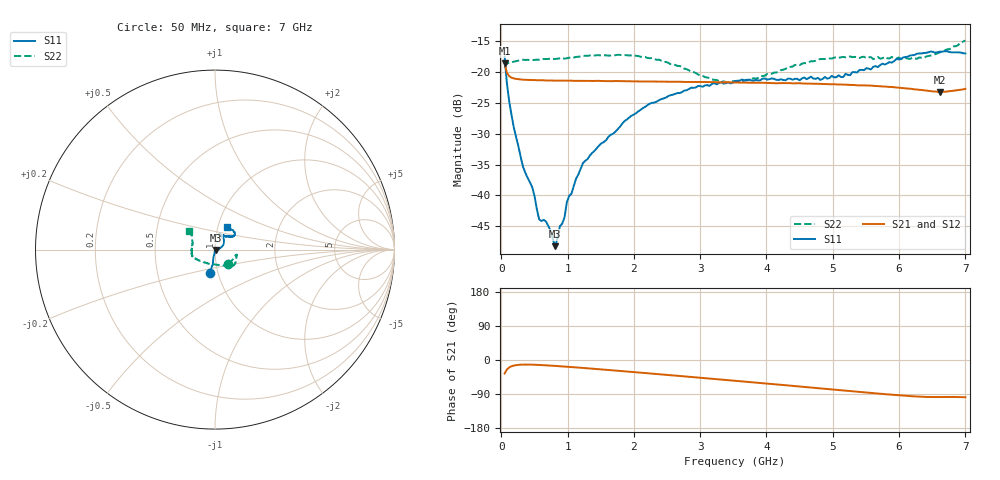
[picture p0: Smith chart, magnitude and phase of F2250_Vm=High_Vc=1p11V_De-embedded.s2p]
! Integrated Device Technology
! Corporate Headquarters
! 6024 Silver Creek Valley Road
! San Jose, CA 95138  USA
! Phone:  1-408-284-8200
! Toll Free:  1-800-223-1366
! Webpage:  http://www.idt.com/
! Timing and RF Division
! 515 Groton Road, Suite 102
! Westford, MA 01886-6024
! Device:  F2250
! Description: Voltage Variable RF Attenuator
! Frequency:  50.0 -  6000.00 MHz
! Package:  3x3 mm Thin QFN Plastic Package: 16 pin
! Ports:  2 RF, 3 DC
!  Pin  1  = GND
!  Pin  2  = NC
!  Pin  3  = RF1  = Port 1
!  Pin  4  = NC
!  Pin  5  = GND
!  Pin  6  = GND
!  Pin  7  = GND
!  Pin  8  = GND
!  Pin  9  = NC
!  Pin 10  = RF2  = Port 2
!  Pin 11  = NC
!  Pin 12  = GND
!  Pin 13  = GND
!  Pin 14  = VCNTRL
!  Pin 15  = VDD
!  Pin 16  = VMODE
! Vcntrl:  1.110 Volts
! Vmode:  +3.300 Volts
! Vdd:  +3.30  Volts
! Current:  1.329 mA
! Data:  The device was measured on a the F2250 evaluation board which has
!  individual transmission lines to the RF pins.  Data was collected
!  using a calibrated network analyzer.  The evaluation board was
!  de-embedded using a TRL calibration technique.
!  The reference plane is the edge of the package pin.
! Misc:  SN 10
!  Action Tracker AT0258
! Date Measured:  2014-11-26
! Date:  2015-10-15  MJV
! Note:
!  Integrated Device Technology supplies this data as a sample of measured
!  data at the package pin for this product.  Your particular data for this
!  product may vary.
!  Data was taken at 25 degrees C.
!  Integrated Device Technology reserves the right to change this data at anytime.
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# GHz S dB R 50
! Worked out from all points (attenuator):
!   201 points, 50 MHz to 7 GHz, reference 50 ohm
!   highest |S21| = -18.58 dB at 50 MHz (marker M1); lowest = -23.2 dB at 6.618 GHz (marker M2)
!   lowest |S11| = -48.2 dB at 814.5 MHz (marker M3), VSWR 1.01, Z = 50.3 - j0.188 ohm
!   |S11| at or under -10 dB: start of sweep to end of sweep
!   |S22| runs from -21.7 to -14.9 dB; largest |S21 - S12| = 0.00041
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0.05  -17.50 -102.6  -18.58 -35.6  -18.58 -35.6  -19.33 -47.2
0.08475  -21.87 -98.4  -20.15 -25.1  -20.14 -25.1  -18.64 -24.3
0.15425  -27.00 -101.4  -20.94 -16.6  -20.93 -16.5  -18.48 -14.7
0.328  -35.36 -98.5  -21.27 -12.1  -21.26 -12.1  -18.03 -13.0
0.467  -38.69 -98.4  -21.32 -12.3  -21.30 -12.3  -18.09 -14.8
0.57125  -43.88 -81.5  -21.35 -13.0  -21.35 -13.1  -18.03 -17.3
0.6755  -44.24 -71.6  -21.39 -14.0  -21.37 -14.0  -17.92 -19.2
0.8145  -48.21 -28.7  -21.42 -15.6  -21.40 -15.6  -17.90 -22.8
0.884  -44.97 -20.2  -21.41 -16.4  -21.41 -16.4  -17.82 -25.0
0.9535  -43.55 -28.2  -21.42 -17.3  -21.42 -17.3  -17.85 -26.1
0.98825  -41.12 -21.4  -21.42 -17.7  -21.43 -17.7  -17.80 -26.8
1.2315  -34.78 2.6  -21.45 -20.9  -21.45 -20.9  -17.40 -31.4
1.857  -27.98 22.0  -21.50 -29.9  -21.52 -29.9  -17.27 -40.2
2.37825  -24.59 34.7  -21.58 -37.5  -21.59 -37.5  -18.01 -48.1
3.1775  -21.94 56.1  -21.67 -49.5  -21.67 -49.6  -21.23 -77.9
3.525  -21.48 66.0  -21.71 -54.9  -21.73 -54.9  -21.54 -102.5
4.7065  -21.09 69.2  -21.92 -73.2  -21.91 -73.2  -18.28 -156.0
5.15825  -20.81 52.9  -22.06 -80.3  -22.05 -80.4  -17.57 -164.7
5.85325  -18.42 37.6  -22.43 -91.1  -22.43 -91.2  -17.83 -179.4
6.3745  -16.94 38.9  -22.98 -97.3  -22.98 -97.3  -17.76 162.3
6.61775  -16.72 44.1  -23.23 -97.5  -23.22 -97.7  -16.82 152.4
7  -17.01 61.9  -22.75 -98.3  -22.76 -98.4  -14.91 145.3
